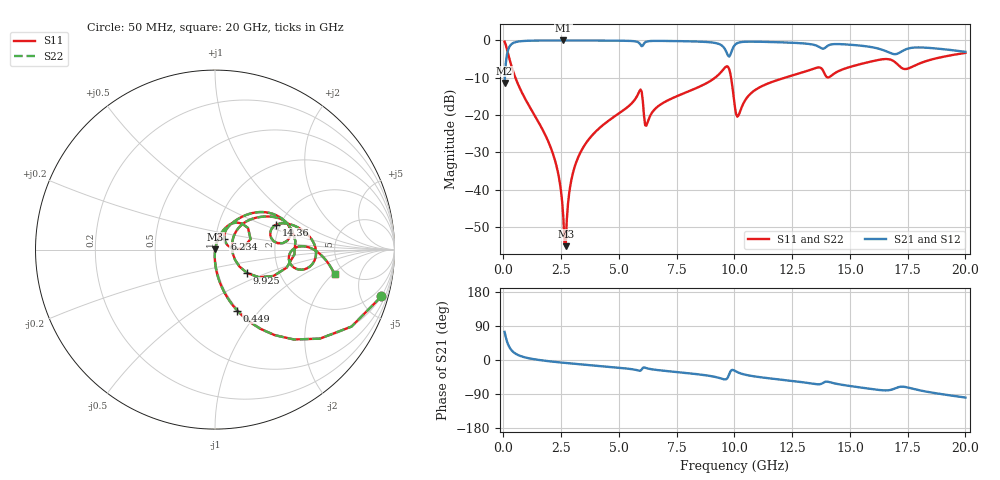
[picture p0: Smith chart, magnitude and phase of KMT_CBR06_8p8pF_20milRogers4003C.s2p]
! Data measured by Modelithics Inc. support@modelithics.com 813-866-6335
! KEMET CBR0603 8.8pF, Pad Width= 0.851mm, Pad Length= 0.64mm, Pad Gap= 0.62mm, 20mil Rogers 4003C substrate Data, January 2022
# hz S ma R 50
! 2 Port Network Data from SP1.SP block
! freq  magS11  angS11  magS21  angS21  magS12  angS12  magS22  angS22
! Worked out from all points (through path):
!   401 points, 50 MHz to 20 GHz, reference 50 ohm
!   highest |S21| = -0.01 dB at 2.594 GHz (marker M1); lowest = -11.4 dB at 50 MHz (marker M2)
!   group delay of S21, straight-line fit = 14.5 ps
!   lowest |S11| = -55.1 dB at 2.693 GHz (marker M3), VSWR 1.00, Z = 50.1 + j0.103 ohm
!   |S11| at or under -10 dB: 518.5 MHz to 9.16 GHz (8.641 GHz wide, 179 % of centre); 9.854 GHz to 12.18 GHz (2.324 GHz wide, 21.1 % of centre)
!   |S22| runs from -55.1 to -0.3 dB; largest |S21 - S12| = 0
!   S11 on the Smith chart (normalised r, x): 50 MHz: 0.99, -7.11; 449 MHz: 0.98, -0.77; 6.234 GHz: 1.10, +0.13; 9.925 GHz: 1.38, -0.38; 14.36 GHz: 1.90, +0.61; 20 GHz: 4.13, -2.10
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5e7  0.9632 -15.7  0.2685 74.3  0.2685 74.3  0.9632 -15.7
4.49e8  0.362 -69.9  0.9313 19.9  0.9313 19.9  0.362 -69.9
2.14475e9  0.03026 -92.3  0.9983 -4.4  0.9983 -4.4  0.03026 -92.3
2.444e9  0.01227 -90.6  0.9986 -6.3  0.9986 -6.3  0.01227 -90.6
2.593625e9  0.004207 -79.9  0.9986 -7.2  0.9986 -7.2  0.004207 -79.9
2.693375e9  0.001759 35.6  0.9986 -7.8  0.9986 -7.8  0.001759 35.6
2.992625e9  0.01604 75.7  0.9984 -9.5  0.9984 -9.5  0.01604 75.7
3.391625e9  0.03424 75.9  0.9979 -11.7  0.9979 -11.7  0.03424 75.9
5.885375e9  0.2085 44.3  0.9178 -28.4  0.9178 -28.4  0.2085 44.3
6.2345e9  0.07921 48.6  0.9709 -22.2  0.9709 -22.2  0.07921 48.6
6.73325e9  0.134 60.5  0.9849 -27.0  0.9849 -27.0  0.134 60.5
8.828e9  0.2712 46.7  0.9511 -41.0  0.9511 -41.0  0.2712 46.7
9.626e9  0.4429 13.9  0.7286 -51.2  0.7286 -51.2  0.4429 13.9
9.92525e9  0.2222 -36.1  0.78 -26.1  0.78 -26.1  0.2222 -36.1
1.0025e10  0.1261 -27.3  0.8736 -28.8  0.8736 -28.8  0.1261 -27.3
1.017462e10  0.09858 15.9  0.9324 -33.3  0.9324 -33.3  0.09858 15.9
1.087288e10  0.2141 42.7  0.9618 -43.3  0.9618 -43.3  0.2141 42.7
1.336662e10  0.4115 23.8  0.8825 -62.2  0.8825 -62.2  0.4115 23.8
1.436412e10  0.3669 22.1  0.8936 -62.1  0.8936 -62.1  0.3669 22.1
1.670825e10  0.5581 -6.1  0.6853 -79.6  0.6853 -79.6  0.5581 -6.1
1.74065e10  0.4137 -5.4  0.7563 -71.3  0.7563 -71.3  0.4137 -5.4
2e10  0.6801 -11.6  0.7027 -99.1  0.7027 -99.1  0.6801 -11.6
